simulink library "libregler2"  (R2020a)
settings: Solver=ode45  StartTime=0.0  StopTime=10.0  RelTol=1e-3
libraries: $bdroot x22, simulink x1

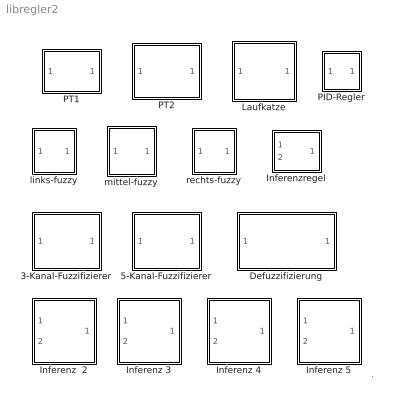
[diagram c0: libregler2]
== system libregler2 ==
  note: .
  3-Kanal-Fuzzifizierer : Subsystem  mask(3-Kanal-Fuzzifizierer){w=1, offset=0}
      mask prompts: w "Breite"; offset "Mittelwert"
      mask help: Erzeugt einen Fuzzy-Wert aus einem scharfen Eingangswert. Verwendet Fuzzyfunktionen mit gleicher Breite. Ausgang: 3 Fuzzy-Signale (zu klein, ok, zu gross) Parameter: (gemeinsame) Breite der Fuzzy-Funktionen
  5-Kanal-Fuzzifizierer : Subsystem  mask(5-Kanal-Fuzzifizierer){w=1, offset=0}
      mask prompts: w "Breite"; offset "Mittelwert"
      mask help: Erzeugt einen Fuzzy-Wert aus einem scharfen Eingangswert. Verwendet Fuzzyfunktionen mit gleicher Breite. Ausgang: 5 Fuzzy-Signale (viel zu klein, zu klein, ok, zu gross, viel zu gross) Parameter: (gemeinsame) Breite der Fuzzy-Funktionen
  Defuzzifizierung : Subsystem  mask(Defuzzification){h=[-2, -1, 0, 1, 2]}
      mask prompts: h "Positionen"
      mask help: Defuzzifiziert das (Vektor-)Eingangssignal nach der Schwerpunktmethode fuer Singletons. Einzugeben sind die Werte, die den unscharfen Eingaengen bei Vollausschlag entsprechen.
  Inferenz  2 : Subsystem  mask(Inferenz 2){M=[1 1 1; 1 1 2 ; 2 2 1]}
      mask prompts: M "Matrix"
      mask help: Erzeugt aus zwei unscharfen Eingaengen einen unscharfen 2-Kanal-Ausgang, verwendet das SUM-PROD-Verfahren mit Singletons. Parameter: M Regelmatrix mit allen Wenn-dann-Beziehungen Eingang E1 bezeichnet die Spalten, E2 die Zeilen von M Elemente von M haben die Werte 1, 2
  Inferenz 3 : Subsystem  mask(Inferenz 3){M=[3 2 1 1 1; 3 3 2 1 1; 3 3 3 2 1]}
      mask prompts: M "Matrix"
      mask help: Erzeugt aus zwei unscharfen Eingaengen einen unscharfen 3-Kanal-Ausgang, verwendet das SUM-PROD-Verfahren mit Singletons. Parameter: M Regelmatrix mit allen Wenn-dann-Beziehungen Eingang E1 bezeichnet die Spalten, E2 die Zeilen von M Elemente von M haben die Werte 1, 2, 3
  Inferenz 4 : Subsystem  mask(Inferenz 4){M=[2 1 1; 3 3 2 ; 4 3 3]}
      mask prompts: M "Matrix"
      mask help: Erzeugt aus zwei unscharfen Eingaengen einen unscharfen 4-Kanal-Ausgang, verwendet das SUM-PROD-Verfahren mit Singletons. Parameter: M Regelmatrix mit allen Wenn-dann-Beziehungen Eingang E1 bezeichnet die Spalten, E2 die Zeilen von M Elemente von M haben die Werte 1, 2, 3, 4
  Inferenz 5 : Subsystem  mask(Inferenz 5){M=[5 4 3; 4 3 2 ; 3 2 1]}
      mask prompts: M "Matrix"
      mask help: Erzeugt aus zwei unscharfen Eingaengen einen unscharfen 5-Kanal-Ausgang, verwendet das SUM-PROD-Verfahren mit Singletons. Parameter: M Regelmatrix mit allen Wenn-dann-Beziehungen Eingang E1 bezeichnet die Spalten, E2 die Zeilen von M Elemente von M haben die Werte 1, 2, 3, 4, 5
  Inferenzregel : Subsystem  mask(Inferenzregel){M=[1,2,3;2,2,2;3,2,1], n=1}
      mask prompts: M "Regelmatrix"; n "Nummer des Ausgangskanals"
      mask help: Erzeugt aus zwei unscharfen Eingaengen einen Kanal eines unscharfen Ausgangs, verwendet das SUM-PROD-Verfahren mit Singletons. Parameter: M Regelmatrix mit allen Wenn-dann-Beziehungen n Nummer des unscharfen Ausgangskanals
  Laufkatze : Subsystem  mask(Laufkatze){mk=100, ml=500, l=3, g=9.81}
      mask prompts: mk "Laufkatzenmasse"; ml "Lastmasse"; l "Seillaenge"; g "Erdbeschleunigung"
      mask help: Modell einer Laufkatze als Regelstrecke
  PID-Regler : Subsystem  mask(PID-Regler){Kp=1, Ki=1, Kd=0}
      mask prompts: Kp "Proportional:"; Ki "Integral:"; Kd "Ableitung:"
      mask help: Regler mit Proportional-, Integral- und Ableitungsanteil.
  PT1 : Subsystem  mask(PT1){T=2, Kp=5}
      mask prompts: T "Verzoegerungszeit T"; Kp "Verstaerkung Kp"
      mask help: Regelstrecke: einfaches Verzoegerungsglied vom PT1-Typ
  PT2 : Subsystem  mask(PT2){D=0.2, om0=1.0, b0=1.0}
      mask prompts: D "Daempfungsgrad"; om0 "Eigenfrequenz"; b0 "Staerke"
      mask help: schwingfaehige Regelstrecke mit Daempfung D Eigenfrequenz om0 Starke b0
  links-fuzzy : Subsystem  mask(Fuzzy-Funktion, linke Ecke){x0=0.3, w=0.7}
      mask help: Fuzzifizierungsfunktion fuer das linke Ende des Intervals. Parameter: x0 max. Eingangswert mit f = 1 w Breite des Abstiegs, f(x0 + w) = 0
  mittel-fuzzy : Subsystem  mask(Fuzzy-Funktion, inneres Intervall){x0=0.3, w=0.5}
      mask prompts: w "xw:"
      mask help: Fuzzifizierungsfunktion fuer ein inneres Interval. Parameter: x0 Eingangswert mit f = 1 w Breite des Anstiegs/Abstiegs, f(x0 - w) = 0 = f(x0 + w)
  rechts-fuzzy : Subsystem  mask(Fuzzy-Funktion, rechte Ecke){x0=0.3, w=0.7}
      mask help: Fuzzifizierungsfunktion fuer das rechte Ende des Intervals. Parameter: x0 min. Eingangswert mit f = 1 w Breite des Anstiegs, f(x0 - w) = 0

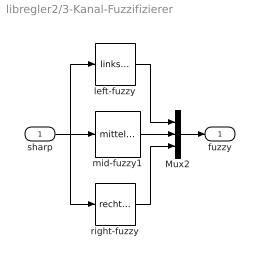
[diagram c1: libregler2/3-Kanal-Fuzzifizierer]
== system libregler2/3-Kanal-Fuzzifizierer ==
  sharp : Inport
  Mux2 : Mux  Inputs=3
  left-fuzzy : $bdroot/links-fuzzy  SystemSampleTime=-1  x0=offset-w  w=w
  mid-fuzzy1 : $bdroot/mittel-fuzzy  SystemSampleTime=-1  x0=offset  w=w
  right-fuzzy : $bdroot/rechts-fuzzy  SystemSampleTime=-1  x0=offset+w  w=w
  fuzzy : Outport
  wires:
  sharp/1 -> right-fuzzy/1, left-fuzzy/1, mid-fuzzy1/1
  Mux2/1 -> fuzzy/1
  mid-fuzzy1/1 -> Mux2/2
  right-fuzzy/1 -> Mux2/3
  left-fuzzy/1 -> Mux2/1

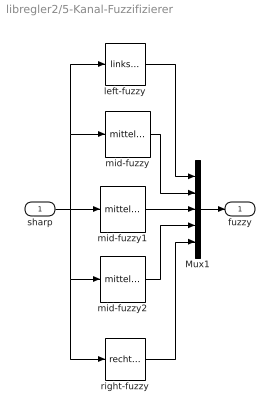
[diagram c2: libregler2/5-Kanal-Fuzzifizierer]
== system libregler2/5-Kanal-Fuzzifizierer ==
  sharp : Inport
  Mux1 : Mux  Inputs=5
  left-fuzzy : $bdroot/links-fuzzy  SystemSampleTime=-1  x0=offset-2*w  w=w
  mid-fuzzy : $bdroot/mittel-fuzzy  SystemSampleTime=-1  x0=offset-w  w=w
  mid-fuzzy1 : $bdroot/mittel-fuzzy  SystemSampleTime=-1  x0=offset  w=w
  mid-fuzzy2 : $bdroot/mittel-fuzzy  SystemSampleTime=-1  x0=offset+w  w=w
  right-fuzzy : $bdroot/rechts-fuzzy  SystemSampleTime=-1  x0=offset+2*w  w=w
  fuzzy : Outport
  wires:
  Mux1/1 -> fuzzy/1
  sharp/1 -> mid-fuzzy/1, left-fuzzy/1, mid-fuzzy2/1, right-fuzzy/1, mid-fuzzy1/1
  right-fuzzy/1 -> Mux1/5
  mid-fuzzy2/1 -> Mux1/4
  mid-fuzzy1/1 -> Mux1/3
  mid-fuzzy/1 -> Mux1/2
  left-fuzzy/1 -> Mux1/1

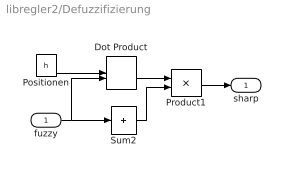
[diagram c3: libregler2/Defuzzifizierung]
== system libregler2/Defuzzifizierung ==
  fuzzy : Inport
  Dot Product : DotProduct
  Positionen : Constant  Value=h
  Product1 : Product  Inputs=*/  InputSameDT=on  SaturateOnIntegerOverflow=on
  Sum2 : Sum  Inputs=+  InputSameDT=on  SaturateOnIntegerOverflow=on
  sharp : Outport
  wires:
  Dot Product/1 -> Product1/1
  fuzzy/1 -> Sum2/1, Dot Product/2
  Positionen/1 -> Dot Product/1
  Sum2/1 -> Product1/2
  Product1/1 -> sharp/1

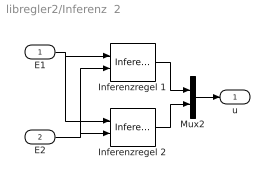
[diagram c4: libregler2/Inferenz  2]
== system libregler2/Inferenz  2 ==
  E1 : Inport
  E2 : Inport  Port=2
  Inferenzregel 1 : $bdroot/Inferenzregel  SystemSampleTime=-1  M=M  n=1
  Inferenzregel 2 : $bdroot/Inferenzregel  SystemSampleTime=-1  M=M  n=2
  Mux2 : Mux  Inputs=2
  u : Outport
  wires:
  E2/1 -> Inferenzregel 2/2, Inferenzregel 1/2
  E1/1 -> Inferenzregel 2/1, Inferenzregel 1/1
  Inferenzregel 1/1 -> Mux2/1
  Mux2/1 -> u/1
  Inferenzregel 2/1 -> Mux2/2

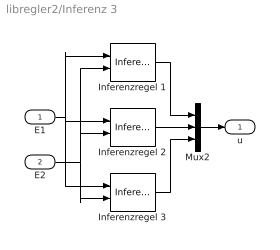
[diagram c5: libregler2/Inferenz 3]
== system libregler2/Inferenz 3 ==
  note: .
  E1 : Inport
  E2 : Inport  Port=2
  Inferenzregel 1 : $bdroot/Inferenzregel  SystemSampleTime=-1  M=M  n=1
  Inferenzregel 2 : $bdroot/Inferenzregel  SystemSampleTime=-1  M=M  n=2
  Inferenzregel 3 : $bdroot/Inferenzregel  SystemSampleTime=-1  M=M  n=3
  Mux2 : Mux  Inputs=3
  u : Outport
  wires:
  E2/1 -> Inferenzregel 3/2, Inferenzregel 1/2, Inferenzregel 2/2
  E1/1 -> Inferenzregel 1/1, Inferenzregel 2/1, Inferenzregel 3/1
  Inferenzregel 3/1 -> Mux2/3
  Inferenzregel 1/1 -> Mux2/1
  Mux2/1 -> u/1
  Inferenzregel 2/1 -> Mux2/2

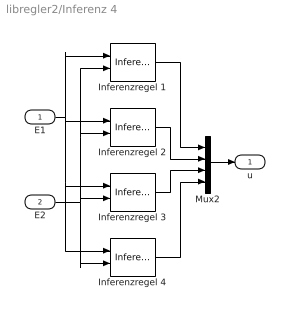
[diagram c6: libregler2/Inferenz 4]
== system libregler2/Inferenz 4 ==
  E1 : Inport
  E2 : Inport  Port=2
  Inferenzregel 1 : $bdroot/Inferenzregel  SystemSampleTime=-1  M=M  n=1
  Inferenzregel 2 : $bdroot/Inferenzregel  SystemSampleTime=-1  M=M  n=2
  Inferenzregel 3 : $bdroot/Inferenzregel  SystemSampleTime=-1  M=M  n=3
  Inferenzregel 4 : $bdroot/Inferenzregel  SystemSampleTime=-1  M=M  n=4
  Mux2 : Mux
  u : Outport
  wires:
  E2/1 -> Inferenzregel 2/2, Inferenzregel 1/2, Inferenzregel 3/2, Inferenzregel 4/2
  E1/1 -> Inferenzregel 2/1, Inferenzregel 1/1, Inferenzregel 3/1, Inferenzregel 4/1
  Inferenzregel 3/1 -> Mux2/3
  Inferenzregel 1/1 -> Mux2/1
  Mux2/1 -> u/1
  Inferenzregel 2/1 -> Mux2/2
  Inferenzregel 4/1 -> Mux2/4

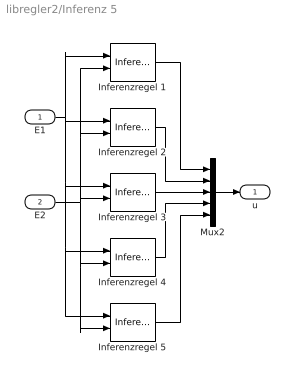
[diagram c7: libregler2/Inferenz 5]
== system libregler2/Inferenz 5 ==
  E1 : Inport
  E2 : Inport  Port=2
  Inferenzregel 1 : $bdroot/Inferenzregel  SystemSampleTime=-1  M=M  n=1
  Inferenzregel 2 : $bdroot/Inferenzregel  SystemSampleTime=-1  M=M  n=2
  Inferenzregel 3 : $bdroot/Inferenzregel  SystemSampleTime=-1  M=M  n=3
  Inferenzregel 4 : $bdroot/Inferenzregel  SystemSampleTime=-1  M=M  n=4
  Inferenzregel 5 : $bdroot/Inferenzregel  SystemSampleTime=-1  M=M  n=5
  Mux2 : Mux  Inputs=5
  u : Outport
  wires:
  E2/1 -> Inferenzregel 3/2, Inferenzregel 4/2, Inferenzregel 5/2, Inferenzregel 1/2, Inferenzregel 2/2
  E1/1 -> Inferenzregel 3/1, Inferenzregel 4/1, Inferenzregel 5/1, Inferenzregel 1/1, Inferenzregel 2/1
  Inferenzregel 3/1 -> Mux2/3
  Inferenzregel 1/1 -> Mux2/1
  Mux2/1 -> u/1
  Inferenzregel 2/1 -> Mux2/2
  Inferenzregel 4/1 -> Mux2/4
  Inferenzregel 5/1 -> Mux2/5

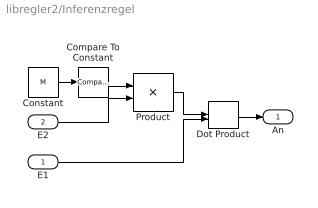
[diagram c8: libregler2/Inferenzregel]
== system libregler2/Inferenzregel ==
  E1 : Inport
  E2 : Inport  Port=2
  Compare To Constant : simulink/Logic and Bit Operations/Compare To Constant  SystemSampleTime=-1  relop===  const=n  LogicOutDataTypeMode=uint8  ZeroCross=off
  Constant : Constant  Value=M
  Dot Product : DotProduct
  Product : Product  Multiplication=Matrix(*)  RndMeth=Zero
  An : Outport
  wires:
  Dot Product/1 -> An/1
  E1/1 -> Dot Product/2
  Product/1 -> Dot Product/1
  E2/1 -> Product/2
  Constant/1 -> Compare To Constant/1
  Compare To Constant/1 -> Product/1

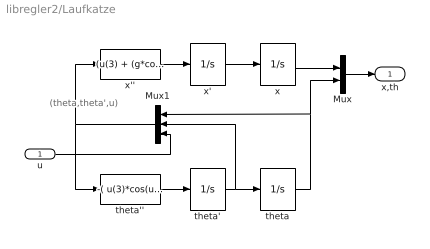
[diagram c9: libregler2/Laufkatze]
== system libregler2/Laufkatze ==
  note: (theta,theta',u)
  u : Inport
  Mux : Mux  Inputs=2
  Mux1 : Mux  Inputs=3
  theta : Integrator
  theta' : Integrator
  theta'' : Fcn  Expr=-( u(3)*cos(u(1)) + (g + l*u(2)^2*cos(u(1)))*ml*sin(u(1)) + g*mk*sin(u(1)) ) / ( (mk + ml*sin(u(1))^2)*l )
  x : Integrator
  x' : Integrator
  x'' : Fcn  Expr=(u(3) + (g*cos(u(1)) + l*u(2)^2)*ml*sin(u(1)))/(mk + ml*sin(u(1))^2)
  x,th : Outport
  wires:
  theta''/1 -> theta'/1
  x''/1 -> x'/1
  u/1 -> Mux1/3
  theta'/1 -> Mux1/2, theta/1
  x'/1 -> x/1
  Mux1/1 -> theta''/1, x''/1
  theta/1 -> Mux1/1, Mux/2
  x/1 -> Mux/1
  Mux/1 -> x,th/1

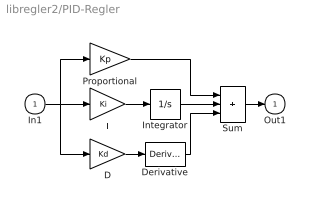
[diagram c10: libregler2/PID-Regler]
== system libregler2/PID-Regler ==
  In1 : Inport
  D : Gain  Gain=Kd  SaturateOnIntegerOverflow=on
  Derivative : Derivative
  I : Gain  Gain=Ki  SaturateOnIntegerOverflow=on
  Integrator : Integrator
  Proportional : Gain  Gain=Kp  SaturateOnIntegerOverflow=on
  Sum : Sum  Inputs=+++  InputSameDT=on  SaturateOnIntegerOverflow=on
  Out1 : Outport  InitialOutput=0
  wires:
  D/1 -> Derivative/1
  Sum/1 -> Out1/1
  In1/1 -> D/1, Proportional/1, I/1
  Derivative/1 -> Sum/3
  Integrator/1 -> Sum/2
  Proportional/1 -> Sum/1
  I/1 -> Integrator/1

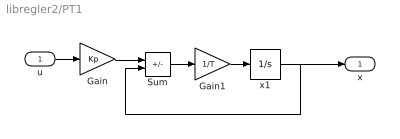
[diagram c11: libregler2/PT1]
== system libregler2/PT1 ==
  u : Inport
  Gain : Gain  Gain=Kp  SaturateOnIntegerOverflow=on
  Gain1 : Gain  Gain=1/T  SaturateOnIntegerOverflow=on
  Sum : Sum  Inputs=+-  SaturateOnIntegerOverflow=on
  x1 : Integrator
  x : Outport
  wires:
  Gain1/1 -> x1/1
  Sum/1 -> Gain1/1
  x1/1 -> Sum/2, x/1
  Gain/1 -> Sum/1
  u/1 -> Gain/1

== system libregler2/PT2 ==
  u : Inport
  Transfer Fcn : TransferFcn  Numerator=[b0]  Denominator=[1 2*D*om0 om0*om0]
  x : Outport
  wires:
  u/1 -> Transfer Fcn/1
  Transfer Fcn/1 -> x/1

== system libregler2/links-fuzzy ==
  In1 : Inport
  1-D Lookup Table : Lookup_n-D  NumberOfTableDimensions=1  BreakpointsForDimension1=[x0 x0+w]  Table=[1 0]  ExtrapMethod=Clip  UseLastTableValue=on  RndMeth=Simplest
  Out1 : Outport
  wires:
  In1/1 -> 1-D Lookup Table/1
  1-D Lookup Table/1 -> Out1/1

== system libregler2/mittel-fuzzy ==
  In1 : Inport
  1-D Lookup Table : Lookup_n-D  NumberOfTableDimensions=1  BreakpointsForDimension1=[x0-w x0 x0+w]  Table=[0 1 0]  ExtrapMethod=Clip  UseLastTableValue=on  RndMeth=Simplest
  Out1 : Outport
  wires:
  In1/1 -> 1-D Lookup Table/1
  1-D Lookup Table/1 -> Out1/1

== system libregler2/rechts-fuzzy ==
  In1 : Inport
  1-D Lookup Table : Lookup_n-D  NumberOfTableDimensions=1  BreakpointsForDimension1=[x0-w x0]  Table=[0 1]  ExtrapMethod=Clip  UseLastTableValue=on  RndMeth=Simplest
  Out1 : Outport
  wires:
  In1/1 -> 1-D Lookup Table/1
  1-D Lookup Table/1 -> Out1/1
